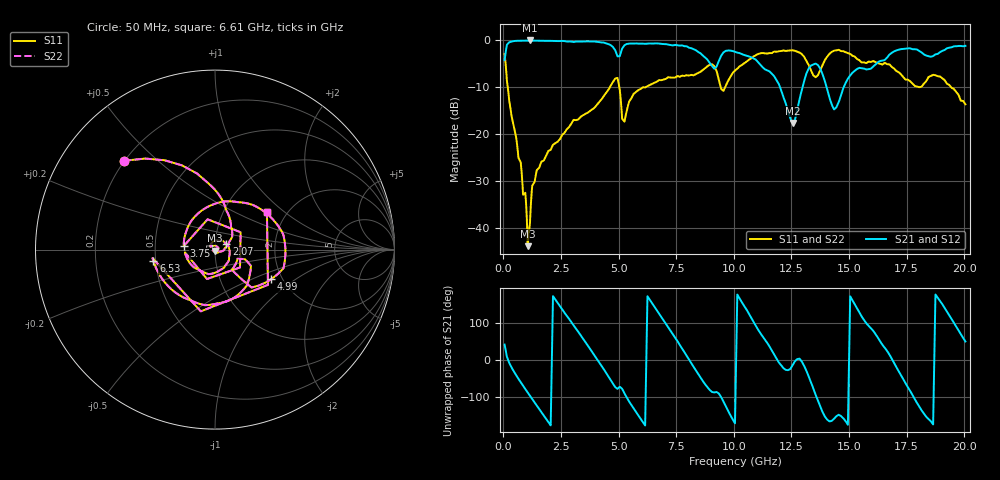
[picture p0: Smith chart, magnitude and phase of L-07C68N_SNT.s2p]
#	mhz	s	ma	r	50
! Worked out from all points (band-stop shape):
!   1001 points, 50 MHz to 20.05 GHz, reference 50 ohm
!   highest |S21| = -0.09 dB at 1.15 GHz (marker M1); lowest = -17.6 dB at 12.55 GHz (marker M2)
!   |S21| within 3 dB of the highest: 82.38 MHz to 4.922 GHz (4.839 GHz wide, 193 % of centre); 5.07 GHz to 8.607 GHz (3.537 GHz wide, 51.7 % of centre)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
!   lowest |S11| = -43.9 dB at 1.05 GHz (marker M3), VSWR 1.01, Z = 49.7 - j0.584 ohm
!   |S11| at or under -10 dB: 186.7 MHz to 4.62 GHz (4.433 GHz wide, 184 % of centre); 5.028 GHz to 6.179 GHz (1.152 GHz wide, 20.6 % of centre); 19.42 GHz to end of sweep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
!   |S22| runs from -43.9 to -2.1 dB; largest |S21 - S12| = 0
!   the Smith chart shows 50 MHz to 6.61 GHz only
!   S11 on the Smith chart (normalised r, x): 50 MHz: 0.20, +0.39; 2.07 GHz: 1.13, +0.07; 3.75 GHz: 0.70, +0.03; 4.99 GHz: 1.76, -0.66; 6.53 GHz: 0.49, -0.07; 6.61 GHz: 1.59, +0.76
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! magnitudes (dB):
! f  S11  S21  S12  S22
! 50 MHz  -3.0  -4.3  -4.3  -3.0
! 1.05 GHz  -43.9  -0.1  -0.1  -43.9
! 1.15 GHz  -39.0  -0.1  -0.1  -39.0
! 1.35 GHz  -30.2  -0.1  -0.1  -30.2
! 2.07 GHz  -23.1  -0.2  -0.2  -23.1
! 3.39 GHz  -16.2  -0.3  -0.3  -16.2
! 3.75 GHz  -15.1  -0.3  -0.3  -15.1
! 4.99 GHz  -9.0  -3.5  -3.5  -9.0
! 5.25 GHz  -17.4  -1.1  -1.1  -17.4
! 6.53 GHz  -9.1  -0.7  -0.7  -9.1
! 6.61 GHz  -9.0  -0.7  -0.7  -9.0
! 6.73 GHz  -8.6  -0.7  -0.7  -8.6
! 9.15 GHz  -5.6  -6.1  -6.1  -5.6
! 9.53 GHz  -10.7  -2.8  -2.8  -10.7
! 10.05 GHz  -6.5  -2.5  -2.5  -6.5
! 11.69 GHz  -2.6  -7.4  -7.4  -2.6
! 12.55 GHz  -2.2  -17.6  -17.6  -2.2
! 13.39 GHz  -6.9  -5.3  -5.3  -6.9
! 14.39 GHz  -2.2  -14.6  -14.6  -2.2
! 15.19 GHz  -3.4  -6.8  -6.8  -3.4
! 16.73 GHz  -5.2  -3.2  -3.2  -5.2
! 20.05 GHz  -13.7  -1.2  -1.2  -13.7
